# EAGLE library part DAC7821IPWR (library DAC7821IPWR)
Digital to Analog Converters - DAC 12-Bit Parallel Inp Multiplying DAC Source: Datasheet
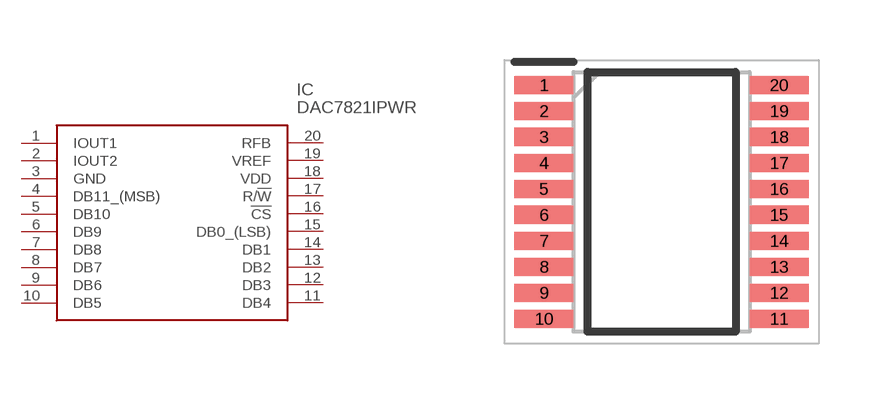
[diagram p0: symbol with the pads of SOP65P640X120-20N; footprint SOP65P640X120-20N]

Designator prefix IC

## DAC7821IPWR (Description: Digital to Analog Converters - DAC 12-Bit Parallel Inp Multiplying DAC; Height: 1.2mm; Manufacturer_Name: Texas Instruments; Manufacturer_Part_Number: DAC7821IPWR; Mouser_Part_Number: 595-DAC7821IPWR; Mouser_Price-Stock: https://www.mouser.co.uk/ProductDetail/Texas-Instruments/DAC7821IPWR?qs=vul0MlC%2Fa1fjuC3krpTQeg%3D%3D)  [SOP65P640X120-20N]
1  IOUT1
2  IOUT2
3  GND
4  DB11_(MSB)
5  DB10
6  DB9
7  DB8
8  DB7
9  DB6
10  DB5
11  DB4
12  DB3
13  DB2
14  DB1
15  DB0_(LSB)
16  !CS
17  R/!W
18  VDD
19  VREF
20  RFB

## Footprint SOP65P640X120-20N (pad centres in mm)
PW (R-PDSO-G20)
smd 1.475 x 0.45: 1 -2.938,2.925; 2 -2.938,2.275; 3 -2.938,1.625; 4 -2.938,0.975; 5 -2.938,0.325; 6 -2.938,-0.325; 7 -2.938,-0.975; 8 -2.938,-1.625; 9 -2.938,-2.275; 10 -2.938,-2.925; 11 2.938,-2.925; 12 2.938,-2.275; 13 2.938,-1.625; 14 2.938,-0.975; 15 2.938,-0.325; 16 2.938,0.325; 17 2.938,0.975; 18 2.938,1.625; 19 2.938,2.275; 20 2.938,2.925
